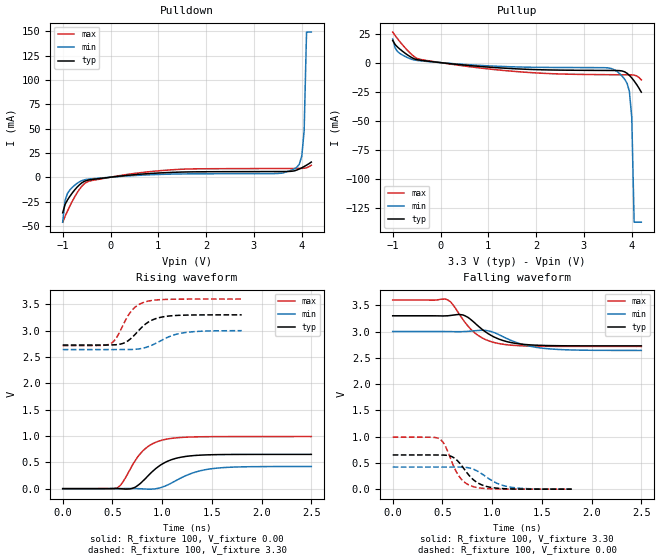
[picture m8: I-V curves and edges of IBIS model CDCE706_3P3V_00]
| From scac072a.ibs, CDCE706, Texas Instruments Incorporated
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|   Model   CDCE706_3P3V_00
[Model]   CDCE706_3P3V_00
Model_type   Output
Polarity   Non-Inverting
Vmeas  =   1.50V
Cref   =   3.00pF
Rref   =   100
Vref   =   0.00V
|Variable   typ   min   max
C_comp   1.452e-12   1.443e-12   1.471e-12
|Variable   typ   min   max
[Voltage range]   3.3   3.0   3.6
|Variable   typ   min   max
[Temperature range]  55   110   -15
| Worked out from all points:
|   slope of the pulldown table from 0 to 0.495 V, typ, clamps not added: 193 ohm
|   slope of the pullup table from 0 to 0.495 V, typ, clamps not added: 235 ohm
|   rising waveform, R_fixture 100, V_fixture 0.00: 20-80 % time 257ps typ, 308ps min, 223ps max; typ from 0 V to 0.651 V
|   falling waveform, R_fixture 100, V_fixture 3.30: 20-80 % time 277ps typ, 322ps min, 248ps max; typ from 3.3 V to 2.73 V
|   rising waveform, R_fixture 100, V_fixture 3.30: 20-80 % time 202ps typ, 253ps min, 166ps max; typ from 2.73 V to 3.3 V
|   falling waveform, R_fixture 100, V_fixture 0.00: 20-80 % time 185ps typ, 228ps min, 151ps max; typ from 0.651 V to 0 V
[Pulldown]
|Voltage   I(typ)   I(min)   I(max)
-1V       -36.59mA   -46.2mA    -46.27mA
-950mV    -27.99mA   -23.78mA   -40.26mA
-900mV    -23.38mA   -16.64mA   -34.82mA
-700mV    -10.27mA   -6.322mA   -16.14mA
-550mV    -4.319mA   -2.758mA   -6.795mA
1.2V      4.792mA    3.102mA    7.329mA
3.5V      5.817mA    3.853mA    8.936mA
3.9V      7.432mA    10.4mA     8.995mA
4V        9.666mA    21.66mA    9.093mA
4.05V     10.97mA    47.82mA    9.256mA
4.1V      12.38mA    149.2mA    9.647mA
4.2V      15.56mA    149.2mA    12.3mA
[Pullup]
|Voltage   I(typ)   I(min)   I(max)
-1V       19.2mA     20.44mA    26.31mA
-950mV    15.6mA     12.64mA    23.37mA
-850mV    11.63mA    7.915mA    18.04mA
-400mV    1.934mA    1.464mA    2.617mA
1.65V     -5.473mA   -3.779mA   -7.908mA
3.45V     -6.735mA   -4.403mA   -10.37mA
3.7V      -6.819mA   -7.894mA   -10.45mA
3.85V     -7.921mA   -14.21mA   -10.49mA
3.95V     -10.93mA   -24.72mA   -10.52mA
4V        -13.17mA   -47.26mA   -10.58mA
4.05V     -15.79mA   -137.5mA   -10.78mA
4.2V      -25.49mA   -137.5mA   -14.9mA
[Ramp]
|Variable   typ   min   max
dV/dt_r  0.1987/1.838e-10   0.1274/2.460e-10   0.3069/1.508e-10
dV/dt_f  0.1730/2.044e-10   0.1084/2.553e-10   0.2668/1.743e-10
R_load  =  50
[Rising Waveform]
R_fixture   =   100
V_fixture   =   0.00
V_fixture_min   =   0.00
V_fixture_max   =   0.00
C_fixture   =   0.00
|Time   V(typ)   V(min)   V(max)
0s        0V         0V         0V
555.6ps   1.867mV    662.9uV    25.02mV
606.1ps   -4.126mV   1.896mV    129.3mV
707.1ps   11.22mV    2.534mV    466.6mV
808.1ps   147.9mV    -4.702mV   722.7mV
909.1ps   337.2mV    -6.685mV   859.2mV
1.01ns    477.9mV    35.14mV    926.5mV
1.187ns   596.4mV    201.4mV    971.4mV
1.49ns    643.7mV    376.6mV    987mV
2.5ns     650.8mV    420.7mV    989.3mV
[Falling Waveform]
R_fixture   =   100
V_fixture   =   3.30
V_fixture_min   =   3.00
V_fixture_max   =   3.60
C_fixture   =   0.00
|Time   V(typ)   V(min)   V(max)
0s        3.3V       3V         3.6V
555.6ps   3.3V       2.999V     3.599V
606.1ps   3.312V     2.998V     3.508V
707.1ps   3.316V     2.999V     3.226V
833.3ps   3.15V      3.016V     2.962V
959.6ps   2.96V      3.014V     2.828V
1.086ns   2.844V     2.924V     2.765V
1.288ns   2.762V     2.765V     2.73V
1.54ns    2.734V     2.676V     2.719V
2.5ns     2.727V     2.641V     2.717V
[Rising Waveform]
R_fixture   =   100
V_fixture   =   3.30
V_fixture_min   =   3.00
V_fixture_max   =   3.60
C_fixture   =   0.00
|Time   V(typ)   V(min)   V(max)
0s        2.726V     2.64V      2.716V
472.7ps   2.728V     2.64V      2.744V
545.5ps   2.734V     2.641V     2.879V
618.2ps   2.767V     2.642V     3.149V
690.9ps   2.859V     2.642V     3.375V
763.6ps   3.001V     2.652V     3.493V
836.4ps   3.131V     2.681V     3.549V
981.8ps   3.252V     2.804V     3.588V
1.2ns     3.293V     2.955V     3.598V
1.8ns     3.3V       2.999V     3.599V
[Falling Waveform]
R_fixture   =   100
V_fixture   =   0.00
V_fixture_min   =   0.00
V_fixture_max   =   0.00
C_fixture   =   0.00
|Time   V(typ)   V(min)   V(max)
0s        651.4mV    421.1mV    990.3mV
472.7ps   650.4mV    421mV      953.5mV
527.3ps   647.6mV    420.6mV    827.8mV
600ps     614.6mV    420.6mV    494.2mV
672.7ps   497.6mV    420.4mV    230.9mV
745.5ps   315.4mV    412.7mV    101.6mV
818.2ps   168.7mV    375.1mV    44.27mV
945.5ps   51.31mV    227.8mV    10.83mV
1.164ns   6.74mV     46.01mV    1.569mV
1.8ns     448.2uV    599.6uV    611.1uV
